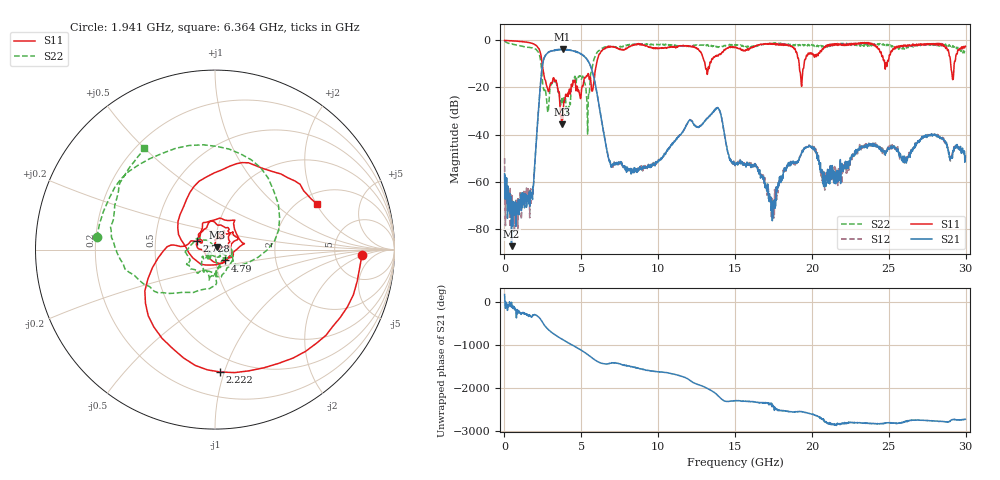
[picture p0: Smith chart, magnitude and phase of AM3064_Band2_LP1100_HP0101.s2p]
# Hz S DB R 50.0
!freq dBS11 angS11 dBS21 angS21 dBS12 angS12 dBS22 angS22
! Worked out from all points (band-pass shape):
!   1600 points, 10 MHz to 29.98 GHz, reference 50 ohm
!   highest |S21| = -3.79 dB at 3.777 GHz (marker M1); lowest = -87.5 dB at 459.8 MHz (marker M2)
!   |S21| within 3 dB of the highest: 2.63 GHz to 5.19 GHz (2.559 GHz wide, 65.5 % of centre)
!   lowest |S11| = -35.7 dB at 3.721 GHz (marker M3), VSWR 1.03, Z = 50.9 + j1.37 ohm
!   |S11| at or under -10 dB: 2.45 GHz to 5.986 GHz (3.536 GHz wide, 83.8 % of centre); 13.05 GHz to 13.35 GHz (304.7 MHz wide, 2.31 % of centre); 19.17 GHz to 19.49 GHz (325.1 MHz wide, 1.68 % of centre)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
!   |S22| runs from -39.8 to -0.3 dB; largest |S21 - S12| = 0.023
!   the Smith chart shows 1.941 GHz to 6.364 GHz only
!   S11 on the Smith chart (normalised r, x): 1.941 GHz: 9.82, -1.67; 2.222 GHz: 0.38, -0.97; 2.728 GHz: 0.81, +0.08; 4.79 GHz: 1.11, -0.14; 6.364 GHz: 2.45, +2.03
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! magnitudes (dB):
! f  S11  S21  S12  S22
! 10 MHz  0.0  -56.7  -50.1  -0.3
! 459.8 MHz  -0.1  -87.5  -77.5  -1.5
! 1.941 GHz  -1.7  -56.4  -56.3  -3.6
! 2.222 GHz  -3.3  -29.0  -28.9  -5.2
! 2.728 GHz  -18.9  -5.8  -5.8  -24.4
! 3.721 GHz  -35.7  -3.8  -3.9  -25.0
! 3.777 GHz  -33.6  -3.8  -3.9  -27.1
! 4.79 GHz  -21.7  -5.1  -5.1  -15.9
! 5.015 GHz  -20.7  -5.9  -5.8  -16.4
! 5.408 GHz  -14.6  -8.4  -8.3  -39.8
! 6.364 GHz  -4.1  -35.8  -35.9  -3.2
! 6.964 GHz  -2.6  -52.8  -52.5  -2.6
! 10 GHz  -3.4  -51.4  -51.1  -1.8
! 13.82 GHz  -6.3  -28.7  -28.7  -2.6
! 15 GHz  -2.8  -53.0  -53.3  -1.8
! 17.5 GHz  -1.6  -70.9  -72.4  -1.2
! 19.33 GHz  -19.5  -47.5  -47.8  -2.1
! 19.99 GHz  -5.4  -45.4  -45.3  -1.8
! 20.83 GHz  -3.1  -57.5  -63.6  -2.3
! 25 GHz  -8.1  -45.9  -45.4  -1.8
! 29.18 GHz  -16.6  -46.8  -47.3  -2.3
! 29.98 GHz  -2.4  -49.2  -50.0  -4.7
